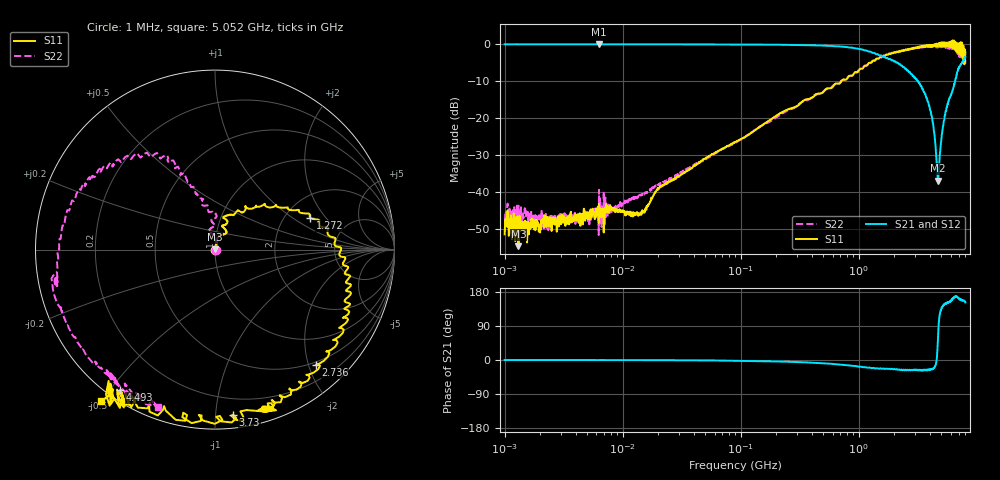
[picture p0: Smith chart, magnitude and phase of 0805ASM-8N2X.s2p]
!s-Parameter Generated by FASTRON Sdn. Bhd.
!FASTRON P/N : 0805ASM-8N2X
!Keysight Technologies: E5071C_MY46733604_B.14.02
!Date: Fri Jun 19 14:47:10 2026
!Version  :Rev00  Fri Jun 19 14:47:10 2026
!Data & Calibration Information:
!Freq  S11:SOLT2(ON)  S21:SOLT2(ON)  S12:SOLT2(ON)  S22:SOLT2(ON)
!PortZ  Port1:50+j0  Port2:50+j0
!When reading reference impedance value at option line is always used.
! Remarks : This data is being provided solely for informational purposes.
# Hz S dB R 50
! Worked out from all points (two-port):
!   1601 points, 1 MHz to 8 GHz, reference 50 ohm
!   highest |S21| = 0.02 dB at 6.301 MHz (marker M1); lowest = -36.8 dB at 4.689 GHz (marker M2)
!   |S21| within 3 dB of the highest: start of sweep to 1.483 GHz
!   lowest |S11| = -54.5 dB at 1.31 MHz (marker M3), VSWR 1.00, Z = 50 + j0.186 ohm
!   |S11| at or under -10 dB: start of sweep to 711.4 MHz
!   |S22| runs from -51.5 to -0.5 dB; largest |S21 - S12| = 0.016
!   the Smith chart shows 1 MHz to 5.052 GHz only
!   S11 on the Smith chart (normalised r, x): 1 MHz: 1.01, -0.00; 1.272 GHz: 2.74, +1.41; 2.736 GHz: 0.45, -2.12; 3.73 GHz: 0.09, -1.11; 4.493 GHz: 0.04, -0.53; 5.052 GHz: -0.03, -0.50
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1000000  -51.30 -19.2  -0.05 -0.1  -0.04 -0.1  -46.80 -3.1
1310238  -54.50 99.1  -0.09 0.2  -0.07 -0.1  -43.60 -22.7
2248791  -48.60 10.0  -0.04 -0.2  -0.06 -0.1  -48.10 11.3
4479405  -47.20 22.1  -0.05 -0.1  -0.05 -0.2  -47.30 28.2
6301378  -43.00 32.8  0.02 -0.2  -0.03 -0.2  -39.30 40.3
1.414737e7  -45.40 61.5  -0.04 -0.3  -0.06 -0.4  -40.70 49.7
2.00676e7  -38.90 62.0  -0.05 -0.5  -0.06 -0.4  -38.00 66.9
8.994653e7  -26.40 77.7  -0.08 -1.9  -0.09 -1.9  -26.60 80.9
4.006501e8  -14.50 75.0  -0.30 -7.0  -0.31 -7.0  -14.30 87.8
1.272209e9  -5.03 18.4  -2.14 -21.3  -2.14 -21.4  -4.96 118.0
1.7949e9  -2.62 -7.2  -4.06 -23.1  -4.06 -23.4  -2.61 138.0
2.736325e9  -1.38 -48.9  -7.86 -27.3  -7.91 -27.3  -1.38 171.0
3.730463e9  -0.67 -83.7  -14.50 -26.6  -14.50 -26.4  -0.73 -158.0
4.135839e9  -0.54 -108.0  -19.30 -23.4  -19.30 -23.6  -0.79 -136.0
4.492594e9  -0.52 -124.0  -28.50 -12.3  -28.50 -12.5  -0.73 -127.0
4.688537e9  -0.43 -125.0  -36.80 57.5  -36.80 57.3  -0.62 -125.0
5.052431e9  0.48 -127.0  -24.40 138.0  -24.40 138.0  -0.61 -110.0
5.472309e9  -0.47 -151.0  -18.10 148.0  -18.10 148.0  -0.68 -74.0
5.995147e9  -0.22 -158.0  -14.00 156.0  -14.00 155.0  -1.30 -66.6
6.57347e9  -1.56 -172.0  -9.84 167.0  -9.80 167.0  -1.70 -21.2
7.306013e9  0.56 165.0  -5.47 159.0  -5.35 159.0  -2.65 -9.4
8e9  -2.22 133.0  -3.41 152.0  -3.31 151.0  -4.31 30.5
